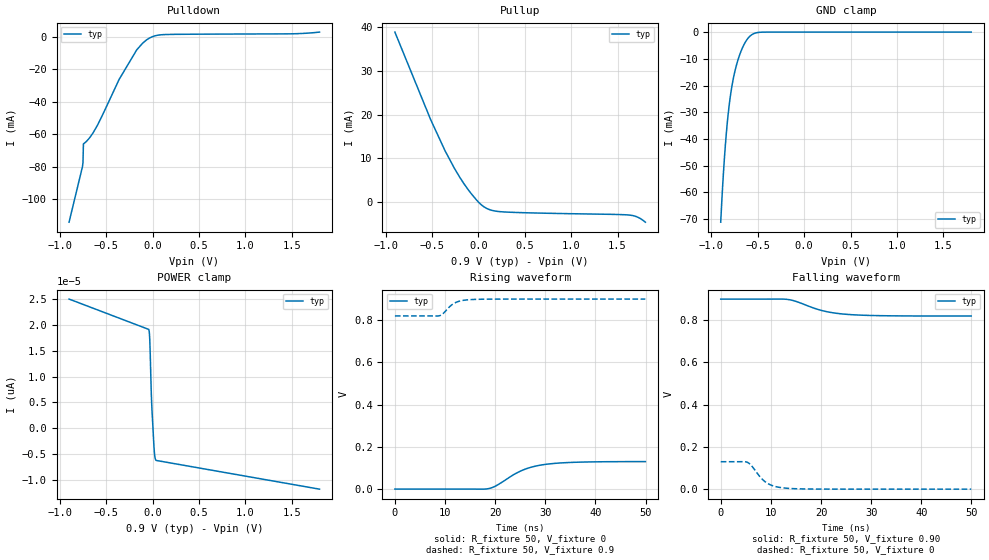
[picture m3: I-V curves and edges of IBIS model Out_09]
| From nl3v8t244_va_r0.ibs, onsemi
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|//////////////////////////////////////////////////////////////////////////////
|//////////////////////////////////////////////////////////////////////////////
[Model] Out_09
Model_type 3-state
Polarity Non-Inverting
Enable Active-Low
Vmeas = 0.45
Vref = 0.9
Rref = 2k
Cref = 15pF
|  variable   typ   min   max
C_comp   5.9pF   5.9pF   5.9pF
|//////////////////////////////////////////////////////////////////////////////
[Temperature Range]   25   125   -40
|//////////////////////////////////////////////////////////////////////////////
[Voltage Range]   0.90V   NA   NA
|//////////////////////////////////////////////////////////////////////////////
[Pulldown Reference]   0V   NA   NA
|//////////////////////////////////////////////////////////////////////////////
[Pullup Reference]   0.90V   NA   NA
|//////////////////////////////////////////////////////////////////////////////
[GND Clamp Reference]   0V   NA   NA
|//////////////////////////////////////////////////////////////////////////////
[POWER Clamp Reference] 0.90V   NA   NA
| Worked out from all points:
|   slope of the pulldown table from 0 to 0.135 V, typ, clamps not added: 105 ohm
|   slope of the pullup table from 0 to 0.135 V, typ, clamps not added: 73.3 ohm
|   GND clamp passes 1 mA (typ) near -0.57 V on its own axis
|   falling waveform, R_fixture 50, V_fixture 0.90: 20-80 % time 6.55ns typ, NA min, NA max; typ from 0.9 V to 0.82 V
|   falling waveform, R_fixture 50, V_fixture 0: 20-80 % time 3.06ns typ, NA min, NA max; typ from 0.13 V to 0 V
|   rising waveform, R_fixture 50, V_fixture 0: 20-80 % time 6.32ns typ, NA min, NA max; typ from 0 V to 0.13 V
|   rising waveform, R_fixture 50, V_fixture 0.9: 20-80 % time 2.34ns typ, NA min, NA max; typ from 0.82 V to 0.9 V
|//////////////////////////////////////////////////////////////////////////////
[Pulldown]
|   Voltage   I(typ)   I(min)   I(max)
-900mV    -114mA     NA         NA
-755mV    -79.79mA   NA         NA
-750mV    -77.44mA   NA         NA
-745mV    -65.81mA   NA         NA
-670mV    -61.49mA   NA         NA
-595mV    -54.58mA   NA         NA
-360mV    -26.24mA   NA         NA
-170mV    -8.078mA   NA         NA
-60mV     -1.806mA   NA         NA
20mV      397.5uA    NA         NA
130mV     1.272mA    NA         NA
1.8V      2.798mA    NA         NA
|//////////////////////////////////////////////////////////////////////////////
[Pullup]
|   Voltage   I(typ)   I(min)   I(max)
-900mV    38.91mA    NA         NA
-515mV    18.89mA    NA         NA
-360mV    11.76mA    NA         NA
-260mV    7.771mA    NA         NA
-150mV    4.012mA    NA         NA
-30mV     716.4uA    NA         NA
50mV      -948.5uA   NA         NA
140mV     -1.873mA   NA         NA
280mV     -2.276mA   NA         NA
1.63V     -2.998mA   NA         NA
1.72V     -3.503mA   NA         NA
1.8V      -4.62mA    NA         NA
|//////////////////////////////////////////////////////////////////////////////
[GND Clamp]
|   Voltage   I(typ)   I(min)   I(max)
-900mV    -71.17mA   NA         NA
-880mV    -58.1mA    NA         NA
-870mV    -52.38mA   NA         NA
-840mV    -38.09mA   NA         NA
-810mV    -27.71mA   NA         NA
-780mV    -20.38mA   NA         NA
-740mV    -13.65mA   NA         NA
-690mV    -7.952mA   NA         NA
-630mV    -3.503mA   NA         NA
-570mV    -1.104mA   NA         NA
-430mV    -13.71uA   NA         NA
1.8V      -3.229pA   NA         NA
|//////////////////////////////////////////////////////////////////////////////
[POWER Clamp]
|   Voltage   I(typ)   I(min)   I(max)
-900mV    24.95pA    NA         NA
-40mV     19.09pA    NA         NA
-35mV     18.58pA    NA         NA
-30mV     17.13pA    NA         NA
-25mV     14.37pA    NA         NA
-15mV     7.634pA    NA         NA
-10mV     5.037pA    NA         NA
-5mV      3.078pA    NA         NA
15mV      -3.465pA   NA         NA
25mV      -5.478pA   NA         NA
40mV      -6.189pA   NA         NA
1.8V      -11.73pA   NA         NA
|//////////////////////////////////////////////////////////////////////////////
|//////////////////////////////////////////////////////////////////////////////
[Ramp]
|  variable   typ   min   max
dV/dt_r   7.800E-02/6.300E-09  7.800E-02/6.300E-09  7.800E-02/6.300E-09
dV/dt_f   4.800E-02/6.300E-09  4.800E-02/6.300E-09  4.800E-02/6.300E-09
R_load = 50
|//////////////////////////////////////////////////////////////////////////////
[Falling Waveform]
R_fixture = 50
V_fixture = 0.90
C_fixture = 0p
|   time   V(typ)   V(min)   V(max)
0s        900mV      NA         NA
12ns      900.2mV    NA         NA
13.2ns    898.8mV    NA         NA
15ns      889.2mV    NA         NA
18.6ns    857.2mV    NA         NA
20.4ns    844.6mV    NA         NA
22.8ns    833.8mV    NA         NA
25.8ns    826.8mV    NA         NA
33.6ns    821.1mV    NA         NA
49.95ns   820mV      NA         NA
|//////////////////////////////////////////////////////////////////////////////
[Falling Waveform]
R_fixture = 50
V_fixture = 0
C_fixture = 0p
|   time   V(typ)   V(min)   V(max)
0s        130mV      NA         NA
4.65ns    130.2mV    NA         NA
5.25ns    127.7mV    NA         NA
6ns       114.7mV    NA         NA
7.8ns     59.55mV    NA         NA
9ns       32.71mV    NA         NA
10.5ns    15.27mV    NA         NA
12.6ns    5.671mV    NA         NA
18.55ns   558.6uV    NA         NA
49.95ns   0V         NA         NA
|//////////////////////////////////////////////////////////////////////////////
[Rising Waveform]
R_fixture = 50
V_fixture = 0
C_fixture = 0p
|   time   V(typ)   V(min)   V(max)
0s        0V         NA         NA
18.3ns    680.3uV    NA         NA
20.1ns    14.65mV    NA         NA
23.7ns    68.44mV    NA         NA
25.2ns    86.8mV     NA         NA
27ns      102.4mV    NA         NA
29.1ns    113.6mV    NA         NA
32.1ns    122.1mV    NA         NA
36ns      126.9mV    NA         NA
49.95ns   130mV      NA         NA
|//////////////////////////////////////////////////////////////////////////////
[Rising Waveform]
R_fixture = 50
V_fixture = 0.9
C_fixture = 0p
|   time   V(typ)   V(min)   V(max)
0s        820mV      NA         NA
8.85ns    820.8mV    NA         NA
9.15ns    823.3mV    NA         NA
9.45ns    828mV      NA         NA
11.1ns    867.7mV    NA         NA
12ns      882.2mV    NA         NA
13.2ns    891.9mV    NA         NA
15ns      897.3mV    NA         NA
20.15ns   899.8mV    NA         NA
49.95ns   900mV      NA         NA
